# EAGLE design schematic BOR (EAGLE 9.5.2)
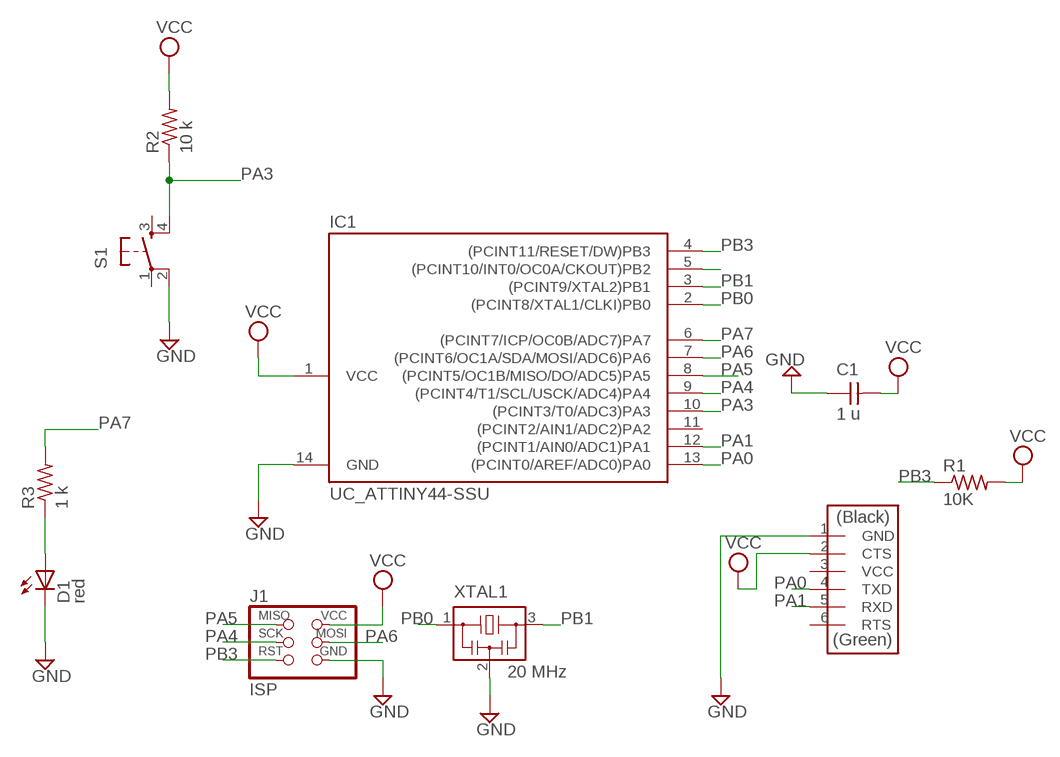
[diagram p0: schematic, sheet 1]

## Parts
C1  1 u  CAP_UNPOLARIZEDFAB  [C1206FAB]
D1  red  LEDFAB1206  [LED1206FAB]
IC1  UC_ATTINY44-SSU  [SOIC14]
J1  ISP  CONN_03X2_AVRISPSMD  [2X03SMD]
J2  FTDI  CONN_06_FTDI-SMD-HEADER  [1X06SMD]
R1  10K  R1206FAB  [R1206FAB]
R2  10 k  R1206FAB  [R1206FAB]
R3  1 k  R1206FAB  [R1206FAB]
S1  SW_SWITCH_TACTILE_6MM6MM_SWITCH  [6MM_SWITCH]
XTAL1  20 MHz  XTAL_RESONATOR  [EFOBM]

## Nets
GND: C1.1 D1.2(C) IC1.14(GND) J1.6(GND) J2.1(GND) S1.2(P1) XTAL1.2
N$1: D1.1(A) R3.1
PA0: IC1.13((PCINT0/AREF/ADC0)PA0) J2.4(TXD)
PA1: IC1.12((PCINT1/AIN0/ADC1)PA1) J2.5(RXD)
PA3: IC1.10((PCINT3/T0/ADC3)PA3) R2.1 S1.4(S1)
PA4: IC1.9((PCINT4/T1/SCL/USCK/ADC4)PA4) J1.3(SCK)
PA5: IC1.8((PCINT5/OC1B/MISO/DO/ADC5)PA5) J1.1(MISO)
PA6: IC1.7((PCINT6/OC1A/SDA/MOSI/ADC6)PA6) J1.4(MOSI)
PA7: IC1.6((PCINT7/ICP/OC0B/ADC7)PA7) R3.2
PB0: IC1.2((PCINT8/XTAL1/CLKI)PB0) XTAL1.1
PB1: IC1.3((PCINT9/XTAL2)PB1) XTAL1.3
PB2: IC1.5((PCINT10/INT0/OC0A/CKOUT)PB2)
PB3: IC1.4((PCINT11/RESET/DW)PB3) J1.5(RST) R1.1
VCC: C1.2 IC1.1(VCC) J1.2(VCC) J2.2(CTS) R1.2 R2.2
Unconnected: IC1.11((PCINT2/AIN1/ADC2)PA2) J2.3(VCC) J2.6(RTS) S1.1(P) S1.3(S)

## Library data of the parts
C1 = eagle_fab:CAP_UNPOLARIZED
D1 = eagle_fab:LED: LED
IC1 = eagle_fab:UC_ATTINY44
J1 = eagle_fab:CONN_03X2_AVRISP
J2 = eagle_fab:CONN_06_FTDI-SMD-HEADER
R1-R3 = eagle_fab:R: Resistor (US Symbol)
S1 = eagle_fab:SW_SWITCH_TACTILE_6MM: OMRON SWITCH
XTAL1 = eagle_fab:XTAL_RESONATOR

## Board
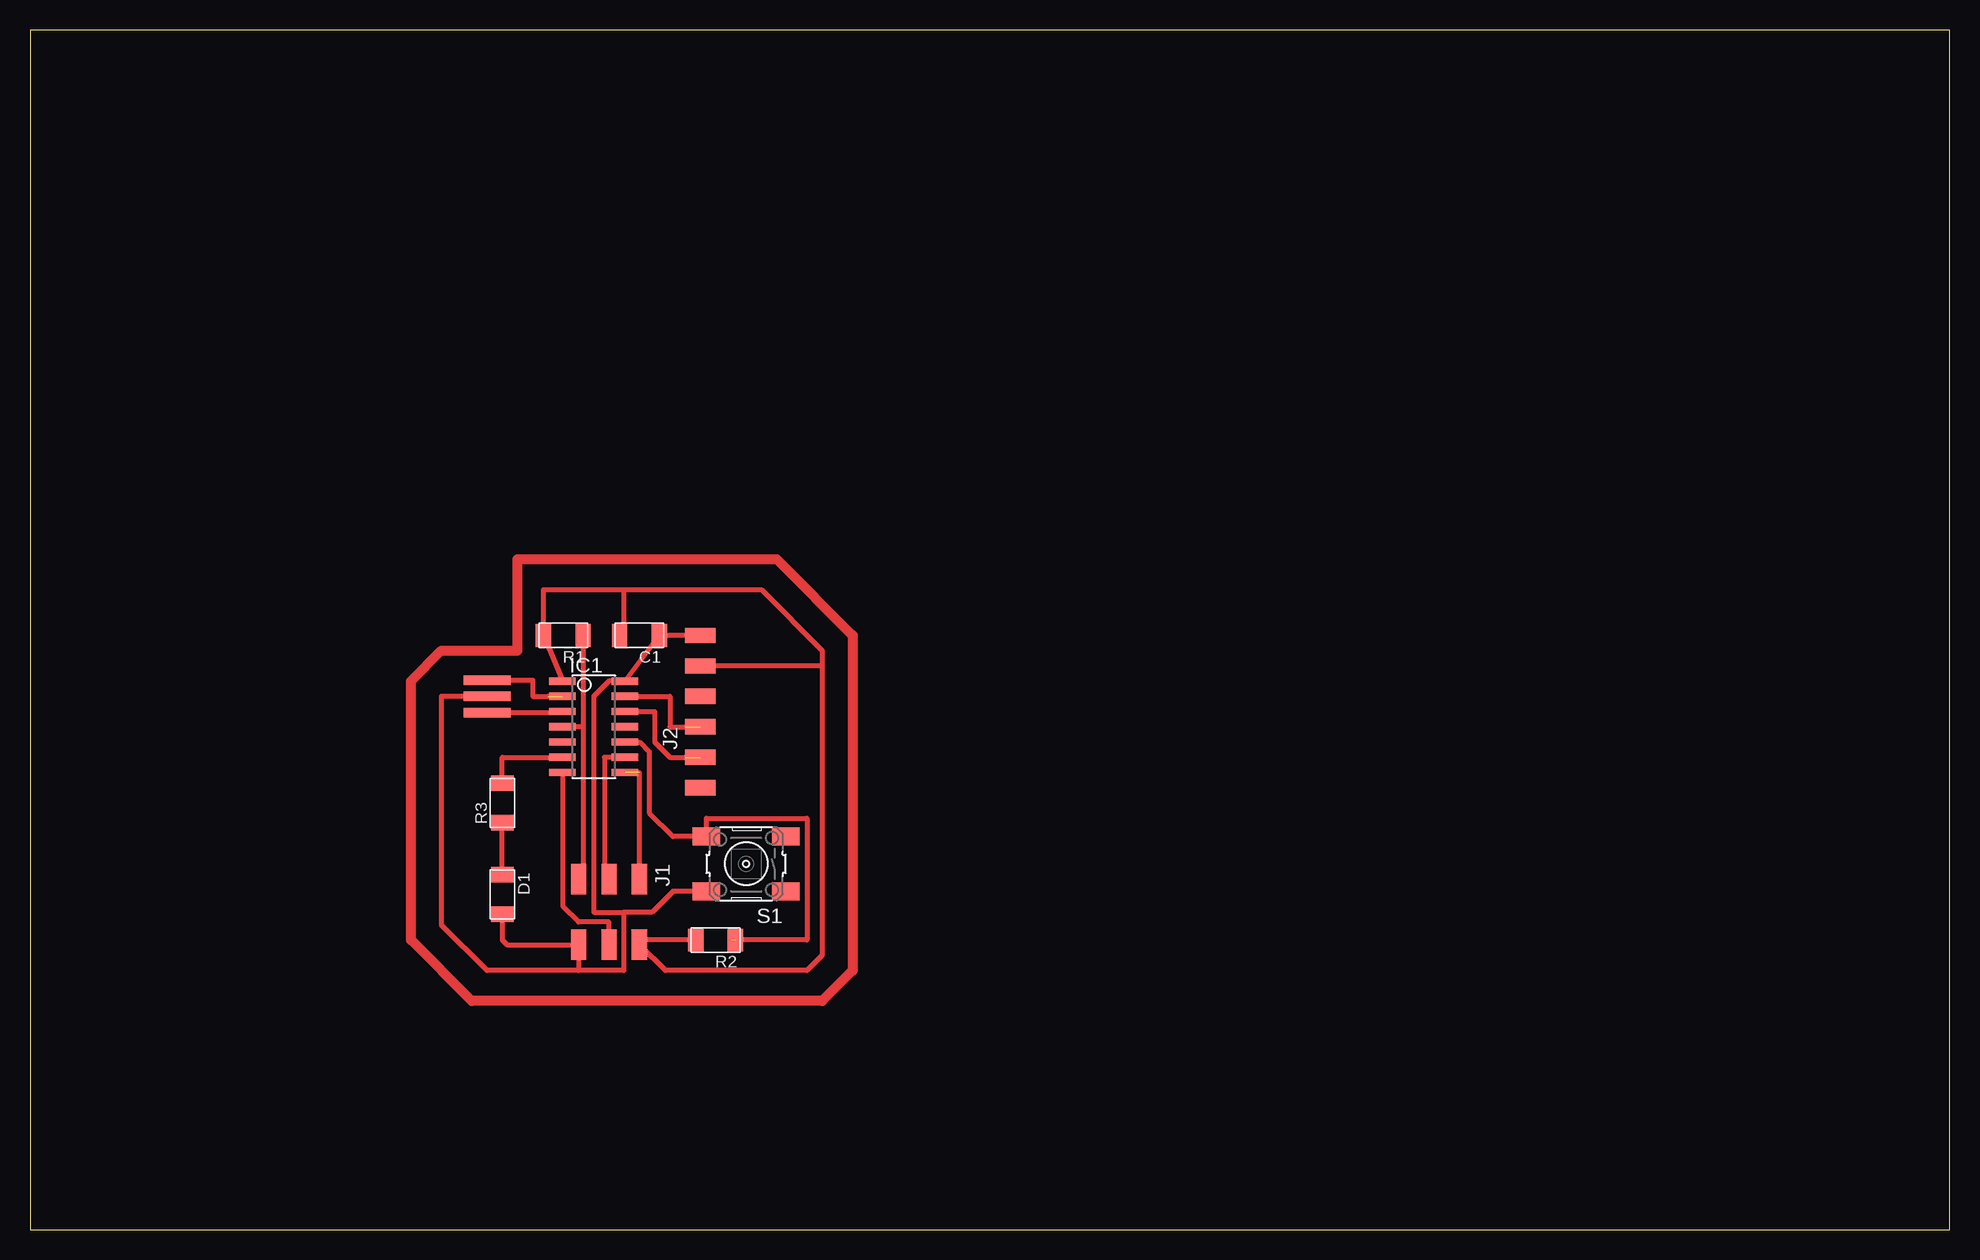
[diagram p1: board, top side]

Size 160 x 100 mm. Coordinates in mm from the lower left corner, seen from the top.
Outline: 0,0 160,0 160,100 0,100 0,0
Copper layers (1*16): Top 0.035mm / dielectric 1.5mm / Bottom 0.035mm
Design rules "default *": minimum track width 10mil, minimum drill 32mil, track to track 16mil, track to pad 16mil, pad to pad 16mil, via to via 16mil, smd to smd 6mil, copper to edge 16mil, drill to drill 16mil, minimum pad ring 10mil, minimum via ring 8mil, stop-mask expansion 4mil, vias tented up to drill 0mil, thermal gap 16mil

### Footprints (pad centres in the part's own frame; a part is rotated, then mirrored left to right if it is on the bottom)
C1206FAB = smd 1.27 x 1.905: 1 -1.651,0; 2 1.651,0
LED1206FAB = smd 1.27 x 1.905: 1 -1.651,0; 2 1.651,0
SOIC14 = smd 0.61 x 2.21: 1 -3.81,-2.603; 2 -2.54,-2.603; 3 -1.27,-2.603; 4 0,-2.603; 5 1.27,-2.603; 6 2.54,-2.603; 7 3.81,-2.603; 8 3.81,2.603; 9 2.54,2.603; 10 1.27,2.603; 11 0,2.603; 12 -1.27,2.603; 13 -2.54,2.603; 14 -3.81,2.603
2X03SMD = smd 2.54 x 1.27: 1 -2.54,2.54; 2 2.92,2.54; 3 -2.54,0; 4 2.92,0; 5 -2.54,-2.54; 6 2.92,-2.54
1X06SMD = smd 2.54 x 1.27: 1 0,6.35; 2 0,3.81; 3 0,1.27; 4 0,-1.27; 5 0,-3.81; 6 0,-6.35
R1206FAB = smd 1.27 x 1.905: 1 -1.651,0; 2 1.651,0
6MM_SWITCH = smd 2.286 x 1.524: 1 -3.302,2.286; 2 3.302,2.286; 3 -3.302,-2.286; 4 3.302,-2.286
EFOBM = smd 0.8 x 3.9: 1 -1.35,0; 2 0,0; 3 1.35,0

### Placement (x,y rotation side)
C1  50.8,49.53 180 top
D1  39.37,27.94 270 top
IC1  46.99,41.91 270 top
J1  48.26,26.67 270 top
J2  55.88,43.18 0 top
R1  44.45,49.53 180 top
R2  57.15,24.13 180 top
R3  39.37,35.56 90 top
S1  59.69,30.48 180 top
XTAL1  38.1,44.45 270 top

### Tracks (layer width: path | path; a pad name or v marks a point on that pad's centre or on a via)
GND
  Top 0.406: J2.1 C1.1 IC1.14 48.26,45.72 46.99,44.45 46.99,26.44 49.51,26.44 | 49.51,26.44 49.51,21.59 45.72,21.59 | 45.72,21.59 38.1,21.59 34.29,25.4 34.29,44.45 XTAL1.2 | S1.2 53.59,28.19 51.84,26.44 49.51,26.44 | D1.2 39.37,24.13 39.75,23.75 J1.6 45.72,21.59
N$1
  Top 0.406: D1.1 R3.1
N$2
  Top 0.813: 40.64,55.88 62.23,55.88 68.58,49.53 68.58,21.59 66.04,19.05 36.83,19.05 31.75,24.13 31.75,45.72 34.29,48.26 40.64,48.26 40.64,55.88
PA0  (1 unrouted)
  Top 0.406: IC1.13 53.34,44.45 53.34,41.91 54.61,41.91
PA1  (1 unrouted)
  Top 0.406: IC1.12 52.07,43.18 52.07,40.64 53.34,39.37 54.61,39.37
PA3  (1 unrouted)
  Top 0.406: 58.42,24.13 64.77,24.13 64.77,34.29 56.39,34.29 S1.4 53.59,32.77 51.61,34.75 51.61,39.83 50.8,40.64 IC1.10
PA4
  Top 0.254: 47.95,29.21 J1.3
  Top 0.406: J1.3 47.88,29.21 47.88,39.37 IC1.9
PA5  (1 unrouted)
  Top 0.406: J1.1 50.8,38.1
PA6
  Top 0.406: J1.4 48.26,25.63 45.72,25.63 44.45,26.9 44.45,38.1 IC1.7
PA7
  Top 0.406: R3.2 39.37,39.37 IC1.6
PB0  (1 unrouted)
  Top 0.406: XTAL1.1 41.91,45.8 41.91,44.45 43.18,44.45
PB1
  Top 0.406: XTAL1.3 44.39,43.1 IC1.3
PB3
  Top 0.406: R1.1 46.1,41.91 | 46.1,41.91 IC1.4 | 46.1,41.91 46.1,29.21 J1.5
VCC
  Top 0.406: 49.53,53.34 49.53,49.53 C1.2 | 49.53,53.34 42.8,53.34 R1.2 IC1.1 | 66.04,46.99 J2.2 | 66.04,46.99 66.04,48.26 60.96,53.34 49.53,53.34 | 66.04,46.99 66.04,22.86 64.77,21.59 52.96,21.59 J1.2 51.18,24.13 R2.2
